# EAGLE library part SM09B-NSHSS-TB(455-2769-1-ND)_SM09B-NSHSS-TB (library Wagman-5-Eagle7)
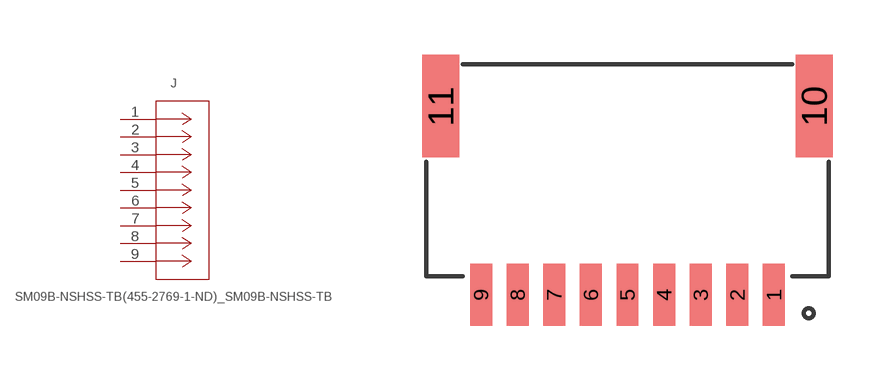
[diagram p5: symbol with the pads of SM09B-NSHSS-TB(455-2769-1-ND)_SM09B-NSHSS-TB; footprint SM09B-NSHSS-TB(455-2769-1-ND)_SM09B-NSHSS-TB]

Designator prefix J

## SM09B-NSHSS-TB(455-2769-1-ND)_SM09B-NSHSS-TB  [SM09B-NSHSS-TB(455-2769-1-ND)_SM09B-NSHSS-TB]
1  1  pas
2  2  pas
3  3  pas
4  4  pas
5  5  pas
6  6  pas
7  7  pas
8  8  pas
9  9  pas

## Footprint SM09B-NSHSS-TB(455-2769-1-ND)_SM09B-NSHSS-TB (pad centres in mm)
smd 0.6 x 1.7: 1 4,0; 2 3,0; 3 2,0; 4 1,0; 5 0,0; 6 -1,0; 7 -2,0; 8 -3,0; 9 -4,0
smd 1 x 2.8: 10 5.1,5.15; 11 -5.1,5.15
